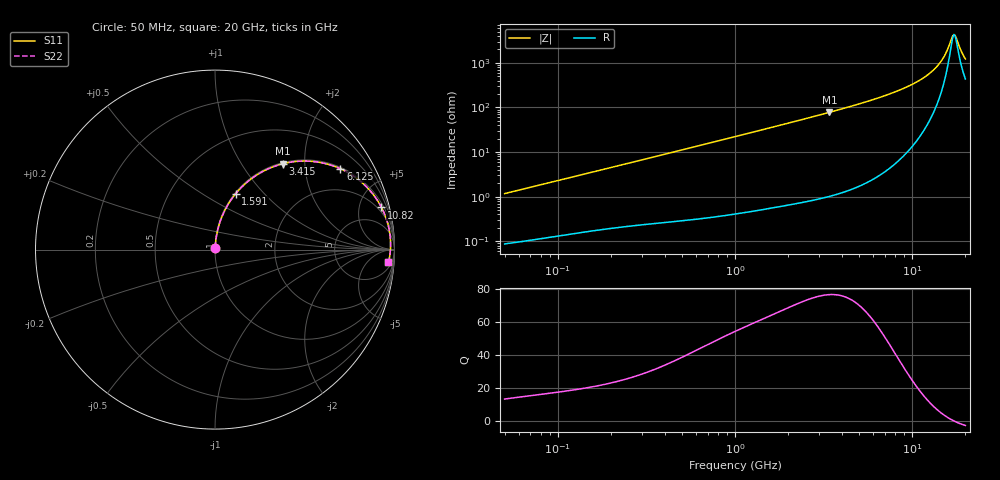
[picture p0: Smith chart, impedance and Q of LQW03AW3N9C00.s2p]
!Murata Part Number: LQW03AW3N9C00
!These Parameters are Measured in Series Mode Connection
!  o--[Z]--o
!Port1  Port2
!  o-------o
!Freq. Start=50[MHz] Stop=20[GHz], 401[Steps]
# Hz S RI R 50
!Freq.(Hz) S11(Real) S11(Imag) S21(Real) S21(Imag) S12(Real) S12(Imag) S22(Real) S22(Imag)
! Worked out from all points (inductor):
!   401 points, 50 MHz to 20 GHz, reference 50 ohm
!   read as one part in series: L = 3.71 nH near 51.52 MHz
!   highest Q = 76.6 at 3.415 GHz (marker M1), where L = 3.63 nH
!   self-resonance near 17.22 GHz
!   S11 on the Smith chart (normalised r, x): 50 MHz: 1.00, +0.02; 1.591 GHz: 1.01, +0.71; 3.415 GHz: 1.02, +1.56; 6.125 GHz: 1.05, +3.07; 10.82 GHz: 1.40, +7.77; 20 GHz: 10, -23
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5e7  0.00101 0.0117  0.999 -0.0117  0.999 -0.0117  0.00101 0.0117
1.364002e8  0.00254 0.031  0.9975 -0.031  0.9975 -0.031  0.00254 0.031
3.721004e8  0.00935 0.0821  0.9906 -0.0821  0.9906 -0.0821  0.00935 0.0821
1e9  0.0503 0.2096  0.9497 -0.2096  0.9497 -0.2096  0.0503 0.2096
1.590961e9  0.1147 0.3109  0.8853 -0.3109  0.8853 -0.3109  0.1147 0.3109
2.083303e9  0.181 0.3779  0.819 -0.3779  0.819 -0.3779  0.181 0.3779
2.728004e9  0.2763 0.4405  0.7237 -0.4405  0.7237 -0.4405  0.2763 0.4405
3.415248e9  0.3791 0.4787  0.6209 -0.4787  0.6209 -0.4787  0.3791 0.4787
4.608136e9  0.5407 0.4915  0.4593 -0.4915  0.4593 -0.4915  0.5407 0.4915
6.125241e9  0.6985 0.4507  0.3015 -0.4507  0.3015 -0.4507  0.6985 0.4507
7.442007e9  0.7947 0.3933  0.2053 -0.3933  0.2053 -0.3933  0.7947 0.3933
9.178299e9  0.8788 0.3105  0.1212 -0.3105  0.1212 -0.3105  0.8788 0.3105
1.082228e10  0.9275 0.235  0.0725 -0.235  0.0725 -0.235  0.9275 0.235
1.257102e10  0.9578 0.1616  0.0422 -0.1616  0.0422 -0.1616  0.9578 0.1616
1.417136e10  0.9722 0.1011  0.0278 -0.1011  0.0278 -0.1011  0.9722 0.1011
1.527346e10  0.9769 0.063  0.0231 -0.063  0.0231 -0.063  0.9769 0.063
1.573793e10  0.9779 0.0478  0.0221 -0.0478  0.0221 -0.0478  0.9779 0.0478
1.670968e10  0.9782 0.0175  0.0218 -0.0175  0.0218 -0.0175  0.9782 0.0175
1.721783e10  0.9775 0.0024  0.0225 -0.0024  0.0225 -0.0024  0.9775 0.0024
1.774144e10  0.9764 -0.0126  0.0236 0.0126  0.0236 0.0126  0.9764 -0.0126
1.912117e10  0.9712 -0.0498  0.0288 0.0498  0.0288 0.0498  0.9712 -0.0498
2e10  0.9665 -0.0718  0.0335 0.0718  0.0335 0.0718  0.9665 -0.0718
